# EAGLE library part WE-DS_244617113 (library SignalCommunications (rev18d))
WE-DS D-SUB-Filter Connectors Bent 90° Characteristics Standard type filtered with 1000 pF High attenuation of more than 40 dB @ 180 MHz Low size: 6.3 mm Rated voltage: 125 VDC Rated current @ 20 ºC: 5 A Withstand voltage: 250 VRMS Insulation resistance: min. 1000 MΩ Operating temperature: –55 ºC to +125 ºC Applications Filtering of interfaces External connection to -printer -sensor -display Details see: http://katalog.we-online.de/en/pbs/D-SUB-Filter Bent 90° Created on 2015-05-04 2015 (C) Wurth Elektronik
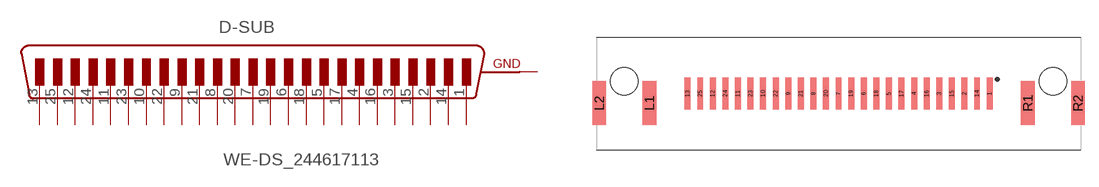
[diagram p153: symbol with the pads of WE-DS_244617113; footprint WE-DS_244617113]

Designator prefix D-SUB

## WE-DS_244617113 (WE-NUMBER: 244617113/25pins_female)  [WE-DS_244617113]
1  13  pas
2  12  pas
3  11  pas
4  10  pas
5  9  pas
6  8  pas
7  7  pas
8  6  pas
9  5  pas
10  4  pas
11  3  pas
12  2  pas
13  1  pas
14  25  pas
15  24  pas
16  23  pas
17  22  pas
18  21  pas
19  20  pas
20  19  pas
21  18  pas
22  17  pas
23  16  pas
24  15  pas
25  14  pas
L1  GND  pwr
L2  GND  pwr
R1  GND  pwr
R2  GND  pwr

## Footprint WE-DS_244617113 (pad centres in mm)
smd 0.65 x 3.5: 1 16.56,0; 2 13.8,0; 3 11.04,0; 4 8.28,0; 5 5.52,0; 6 2.76,0; 7 0,0; 8 -2.76,0; 9 -5.52,0; 10 -8.28,0; 11 -11.04,0; 12 -13.8,0; 13 -16.56,0; 14 15.18,0; 15 12.42,0; 16 9.66,0; 17 6.9,0; 18 4.14,0; 19 1.38,0; 20 -1.38,0; 21 -4.14,0; 22 -6.9,0; 23 -9.66,0; 24 -12.42,0; 25 -15.18,0
smd 1.5 x 4.8: L1 -20.75,-1.05; L2 -26.25,-1.05; R1 20.75,-1.05; R2 26.25,-1.05
hole 3 at -23.5,1.35
hole 3 at 23.5,1.35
